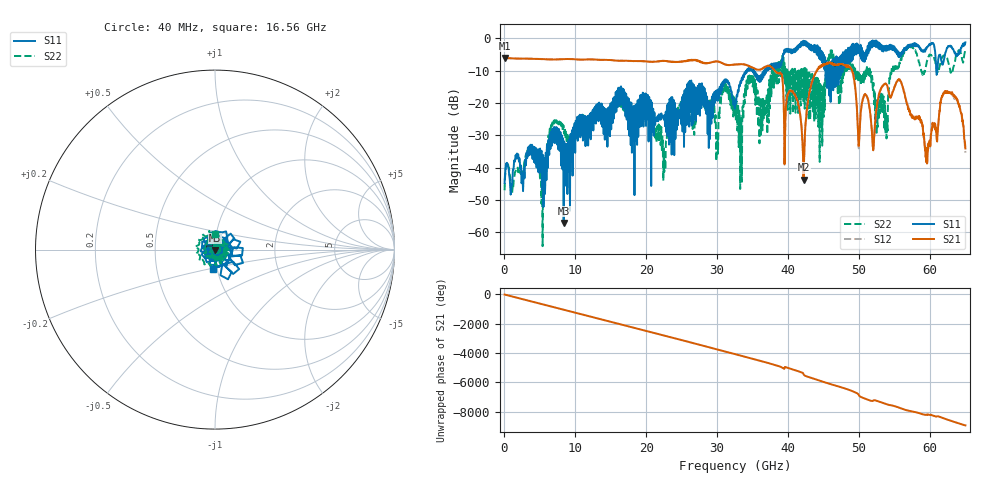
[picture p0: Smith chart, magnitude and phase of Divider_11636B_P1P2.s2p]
! Created Tue Jul 15 20:13:34 2008
# hz S ma R 50
! 2 Port Network Data from blockName block
! freq  magS11  angS11  magS21  angS21  magS12  angS12  magS22  angS22
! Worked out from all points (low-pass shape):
!   1601 points, 40 MHz to 65 GHz, reference 50 ohm
!   highest |S21| = -6.05 dB at 40 MHz (marker M1); lowest = -43.7 dB at 42.18 GHz (marker M2)
!   |S21| within 3 dB of the highest: start of sweep to 35.01 GHz; 44.46 GHz to 48.8 GHz (4.341 GHz wide, 9.31 % of centre)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
!   lowest |S11| = -57.2 dB at 8.363 GHz (marker M3), VSWR 1.00, Z = 50 - j0.138 ohm
!   |S11| at or under -10 dB: start of sweep to 34.19 GHz; 35.19 GHz to 36.58 GHz (1.389 GHz wide, 3.87 % of centre); 36.59716 GHz to 36.73792 GHz (140.8 MHz wide, 0.384 % of centre)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
!   |S22| runs from -64.4 to -2.4 dB; largest |S21 - S12| = 0.021
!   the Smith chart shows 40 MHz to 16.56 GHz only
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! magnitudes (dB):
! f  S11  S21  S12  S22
! 40 MHz  -44.8  -6.1  -6.0  -47.1
! 3.694 GHz  -32.9  -6.3  -6.3  -34.0
! 5.318 GHz  -46.7  -6.4  -6.4  -44.6
! 6.698 GHz  -33.3  -6.5  -6.5  -27.6
! 8.363 GHz  -57.2  -6.4  -6.4  -27.4
! 10.88 GHz  -28.5  -6.6  -6.6  -25.4
! 21.72 GHz  -25.1  -7.1  -7.1  -27.9
! 22.53 GHz  -24.4  -7.0  -7.0  -41.5
! 25.37 GHz  -18.9  -7.0  -7.1  -18.7
! 32.52 GHz  -20.7  -8.0  -8.1  -19.9
! 38.85 GHz  -9.0  -10.7  -10.6  -7.4
! 42.18 GHz  -0.7  -43.7  -42.6  -14.4
! 43.36 GHz  -3.4  -13.6  -13.4  -12.7
! 48.64 GHz  -3.0  -8.8  -8.6  -9.4
! 49.94 GHz  -4.5  -33.3  -33.5  -11.3
! 50.99 GHz  -6.4  -17.6  -17.5  -11.2
! 52.01 GHz  -2.4  -34.7  -33.2  -14.0
! 54.2 GHz  -2.5  -16.7  -16.7  -17.3
! 56.72 GHz  -2.5  -20.0  -19.6  -3.5
! 59.56 GHz  -2.7  -37.1  -35.0  -7.2
! 63.01 GHz  -2.5  -17.3  -17.2  -10.6
! 65 GHz  -1.2  -34.1  -35.4  -3.3
